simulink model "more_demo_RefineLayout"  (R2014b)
settings: Solver=ode45  SolverMode=SingleTasking  StartTime=0.0  StopTime=10.0  RelTol=1e-3

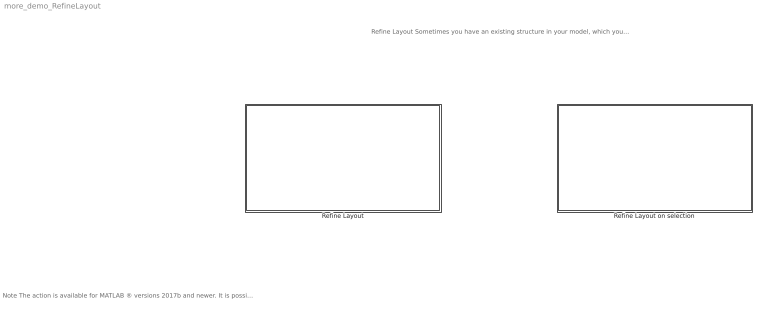
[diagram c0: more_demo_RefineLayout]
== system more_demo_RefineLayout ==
  note: Note The action is available for MATLAB ® versions 2017b and newer. It is possible to set custom parameters for blocks and lines with this action. Simply activate the feature via "Preferences -> Config File" and set "ApplyMoRePreferencesToBlocksAndLines" to true.
  note: Refine Layout Sometimes you have an existing structure in your model, which you would like to preserve, while still improving the layout. This action can be used to create a clean and uniform layout for the current subsystem or selected subarea, while also taking into account the current layout.
  Refine Layout : Subsystem
  Refine Layout on selection : Subsystem

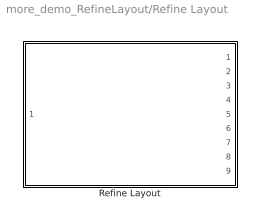
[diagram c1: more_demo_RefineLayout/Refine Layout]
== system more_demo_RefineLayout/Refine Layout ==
  Refine Layout : Subsystem

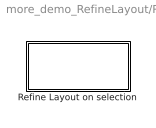
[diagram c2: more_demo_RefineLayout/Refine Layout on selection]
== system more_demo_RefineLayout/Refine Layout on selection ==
  Refine Layout on selection : Subsystem

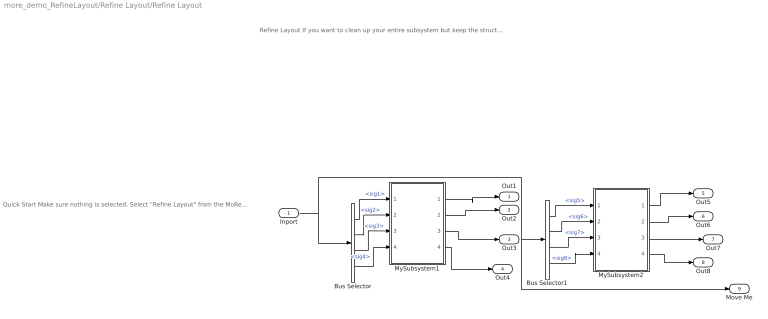
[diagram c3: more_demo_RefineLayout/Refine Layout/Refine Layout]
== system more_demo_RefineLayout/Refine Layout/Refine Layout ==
  note: Refine Layout If you want to clean up your entire subsystem but keep the structure or make some minor adjustments, you can use the Refine Layout action.
  note: Quick Start Make sure nothing is selected. Select "Refine Layout" from the MoRe menu and note the changes. Move the outport bock "Move Me" up over outport block "Out5", reapply the action, and note the changes. If you want, you can undo the changes via the MoRe menu and try "Auto Layout" to see the differences.
  Inport : Inport
  Bus Selector : BusSelector  OutputSignals=sig1,sig2,sig3,sig4
  Bus Selector1 : BusSelector  OutputSignals=sig5,sig6,sig7,sig8
  MySubsystem1 : Subsystem
  MySubsystem2 : Subsystem
  Out1 : Outport
  Out2 : Outport  Port=2
  Out3 : Outport  Port=3
  Out4 : Outport  Port=4
  Out5 : Outport  Port=5
  Out6 : Outport  Port=6
  Out7 : Outport  Port=7
  Out8 : Outport  Port=8
  Move Me : Outport  Port=9
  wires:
  MySubsystem2/3(Out3) -> Out7/1
  Bus Selector/3 -> MySubsystem1/3(In3)  "<sig3>"
  Bus Selector/2 -> MySubsystem1/2(In2)  "<sig2>"
  Bus Selector/4 -> MySubsystem1/4(In4)  "<sig4>"
  MySubsystem2/2(Out2) -> Out6/1
  Bus Selector1/1 -> MySubsystem2/1(In1)  "<sig5>"
  Inport/1 -> Move Me/1, Bus Selector1/1, Bus Selector/1
  Bus Selector1/4 -> MySubsystem2/4(In4)  "<sig8>"
  MySubsystem2/1(Out1) -> Out5/1
  MySubsystem1/1(Out1) -> Out1/1
  Bus Selector/1 -> MySubsystem1/1(In1)  "<sig1>"
  Bus Selector1/2 -> MySubsystem2/2(In2)  "<sig6>"
  MySubsystem1/3(Out3) -> Out3/1
  MySubsystem1/4(Out4) -> Out4/1
  Bus Selector1/3 -> MySubsystem2/3(In3)  "<sig7>"
  MySubsystem1/2(Out2) -> Out2/1
  MySubsystem2/4(Out4) -> Out8/1

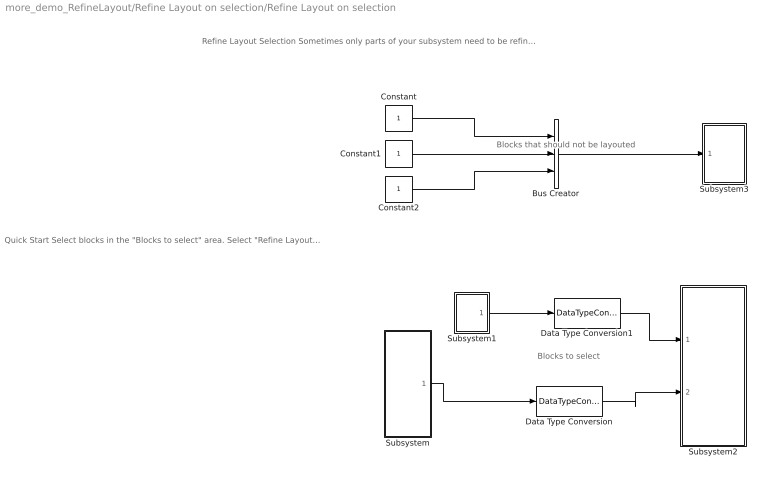
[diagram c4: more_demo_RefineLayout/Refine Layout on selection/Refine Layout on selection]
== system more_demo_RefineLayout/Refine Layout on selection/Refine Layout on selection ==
  note: Refine Layout Selection Sometimes only parts of your subsystem need to be refined. This can also be done with the Refine Layout action.
  note: Quick Start Select blocks in the "Blocks to select" area. Select "Refine Layout Selection" from the MoRe menu and note the changes.
  note: Blocks that should not be layouted
  note: Blocks to select
  Bus Creator : BusCreator  Inputs=3
  Constant : Constant
  Constant1 : Constant
  Constant2 : Constant
  Data Type Conversion : DataTypeConversion
  Data Type Conversion1 : DataTypeConversion
  Subsystem : Subsystem
  Subsystem1 : Subsystem
  Subsystem2 : Subsystem
  Subsystem3 : Subsystem
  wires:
  Subsystem/1(Out1) -> Data Type Conversion/1
  Subsystem1/1(Out1) -> Data Type Conversion1/1
  Data Type Conversion/1 -> Subsystem2/2(In1)
  Data Type Conversion1/1 -> Subsystem2/1(In2)
  Constant/1 -> Bus Creator/1
  Constant2/1 -> Bus Creator/3
  Constant1/1 -> Bus Creator/2
  Bus Creator/1 -> Subsystem3/1(In1)

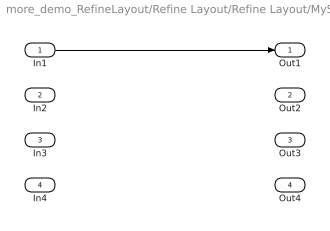
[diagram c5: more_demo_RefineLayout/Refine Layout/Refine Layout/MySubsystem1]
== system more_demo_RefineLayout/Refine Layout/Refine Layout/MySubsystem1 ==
  In1 : Inport
  In2 : Inport  Port=2
  In3 : Inport  Port=3
  In4 : Inport  Port=4
  Out1 : Outport
  Out2 : Outport  Port=2
  Out3 : Outport  Port=3
  Out4 : Outport  Port=4
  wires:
  In1/1 -> Out1/1

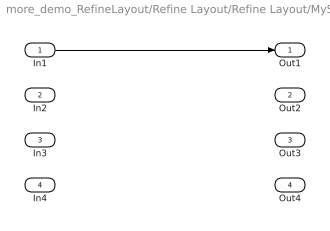
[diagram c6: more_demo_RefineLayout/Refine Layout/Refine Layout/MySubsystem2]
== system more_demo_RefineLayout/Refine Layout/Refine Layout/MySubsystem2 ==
  In1 : Inport
  In2 : Inport  Port=2
  In3 : Inport  Port=3
  In4 : Inport  Port=4
  Out1 : Outport
  Out2 : Outport  Port=2
  Out3 : Outport  Port=3
  Out4 : Outport  Port=4
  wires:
  In1/1 -> Out1/1

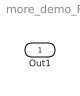
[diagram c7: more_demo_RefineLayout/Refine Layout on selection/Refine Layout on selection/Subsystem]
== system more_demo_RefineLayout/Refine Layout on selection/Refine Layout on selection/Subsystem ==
  Out1 : Outport

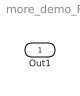
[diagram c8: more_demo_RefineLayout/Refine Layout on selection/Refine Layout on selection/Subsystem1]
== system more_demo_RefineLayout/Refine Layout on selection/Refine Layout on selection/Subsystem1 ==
  Out1 : Outport

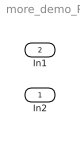
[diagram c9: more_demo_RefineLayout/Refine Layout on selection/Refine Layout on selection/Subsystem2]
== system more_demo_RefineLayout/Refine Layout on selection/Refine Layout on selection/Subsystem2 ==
  In2 : Inport
  In1 : Inport  Port=2

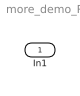
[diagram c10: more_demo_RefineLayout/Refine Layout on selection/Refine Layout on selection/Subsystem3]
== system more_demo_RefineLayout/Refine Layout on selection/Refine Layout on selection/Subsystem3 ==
  In1 : Inport
